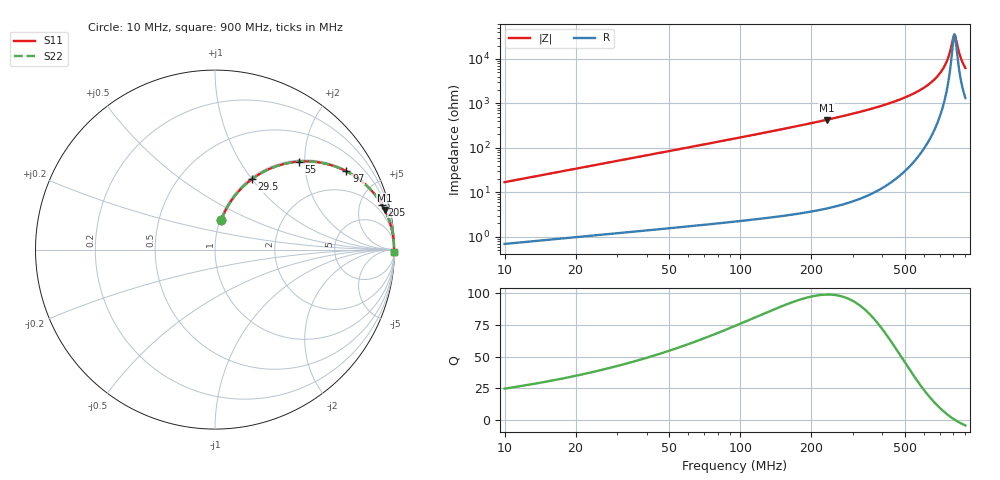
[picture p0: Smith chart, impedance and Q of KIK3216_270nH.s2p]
!version-2
!date-01.2022
!Series
# MHz S RI R 50
!Freq ReS11 ImS11 ReS21 ImS21 ReS12 ImS12 ReS22 ImS22
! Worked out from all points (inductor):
!   595 points, 10 MHz to 900 MHz, reference 50 ohm
!   read as one part in series: L = 269 nH near 13 MHz
!   highest Q = 99.1 at 232 MHz (marker M1), where L = 293 nH
!   self-resonance near 808 MHz
!   S11 on the Smith chart (normalised r, x): 10 MHz: 1.01, +0.34; 29.5 MHz: 1.02, +1.00; 55 MHz: 1.03, +1.87; 97 MHz: 1.04, +3.33; 205 MHz: 1.08, +7.41; 900 MHz: open
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10  0.0341 0.1622  0.9659 -0.1622  0.9659 -0.1622  0.0341 0.1622
19  0.1005 0.2863  0.8995 -0.2863  0.8995 -0.2863  0.1005 0.2863
29.5  0.2052 0.3922  0.7948 -0.3922  0.7948 -0.3922  0.2052 0.3922
55  0.4665 0.4902  0.5335 -0.4902  0.5335 -0.4902  0.4665 0.4902
74.5  0.6156 0.479  0.3844 -0.479  0.3844 -0.479  0.6156 0.479
97  0.7318 0.4364  0.2682 -0.4364  0.2682 -0.4364  0.7318 0.4364
158.5  0.8832 0.3158  0.1168 -0.3158  0.1168 -0.3158  0.8832 0.3158
205  0.9298 0.2504  0.0702 -0.2504  0.0702 -0.2504  0.9298 0.2504
232  0.9461 0.2209  0.0539 -0.2209  0.0539 -0.2209  0.9461 0.2209
307  0.9719 0.16  0.0281 -0.16  0.0281 -0.16  0.9719 0.16
455.5  0.9907 0.0877  0.00933 -0.0877  0.00933 -0.0877  0.9907 0.0877
604  0.9962 0.0431  0.00375 -0.0431  0.00375 -0.0431  0.9962 0.0431
694  0.9973 0.0224  0.00274 -0.0224  0.00274 -0.0224  0.9973 0.0224
727  0.9974 0.0156  0.00263 -0.0156  0.00263 -0.0156  0.9974 0.0156
752.5  0.9974 0.0105  0.00262 -0.0105  0.00262 -0.0105  0.9974 0.0105
775  0.9973 0.00625  0.00266 -0.00625  0.00266 -0.00625  0.9973 0.00625
802  0.9972 0.00127  0.00276 -0.00127  0.00276 -0.00127  0.9972 0.00127
809.5  0.9972 -8.26e-05  0.0028 8.26e-05  0.0028 8.26e-05  0.9972 -8.26e-05
817  0.9972 -0.00142  0.00284 0.00142  0.00284 0.00142  0.9972 -0.00142
838  0.997 -0.00511  0.00299 0.00511  0.00299 0.00511  0.997 -0.00511
854.5  0.9969 -0.00794  0.00312 0.00794  0.00312 0.00794  0.9969 -0.00794
900  0.9964 -0.0155  0.00357 0.0155  0.00357 0.0155  0.9964 -0.0155
